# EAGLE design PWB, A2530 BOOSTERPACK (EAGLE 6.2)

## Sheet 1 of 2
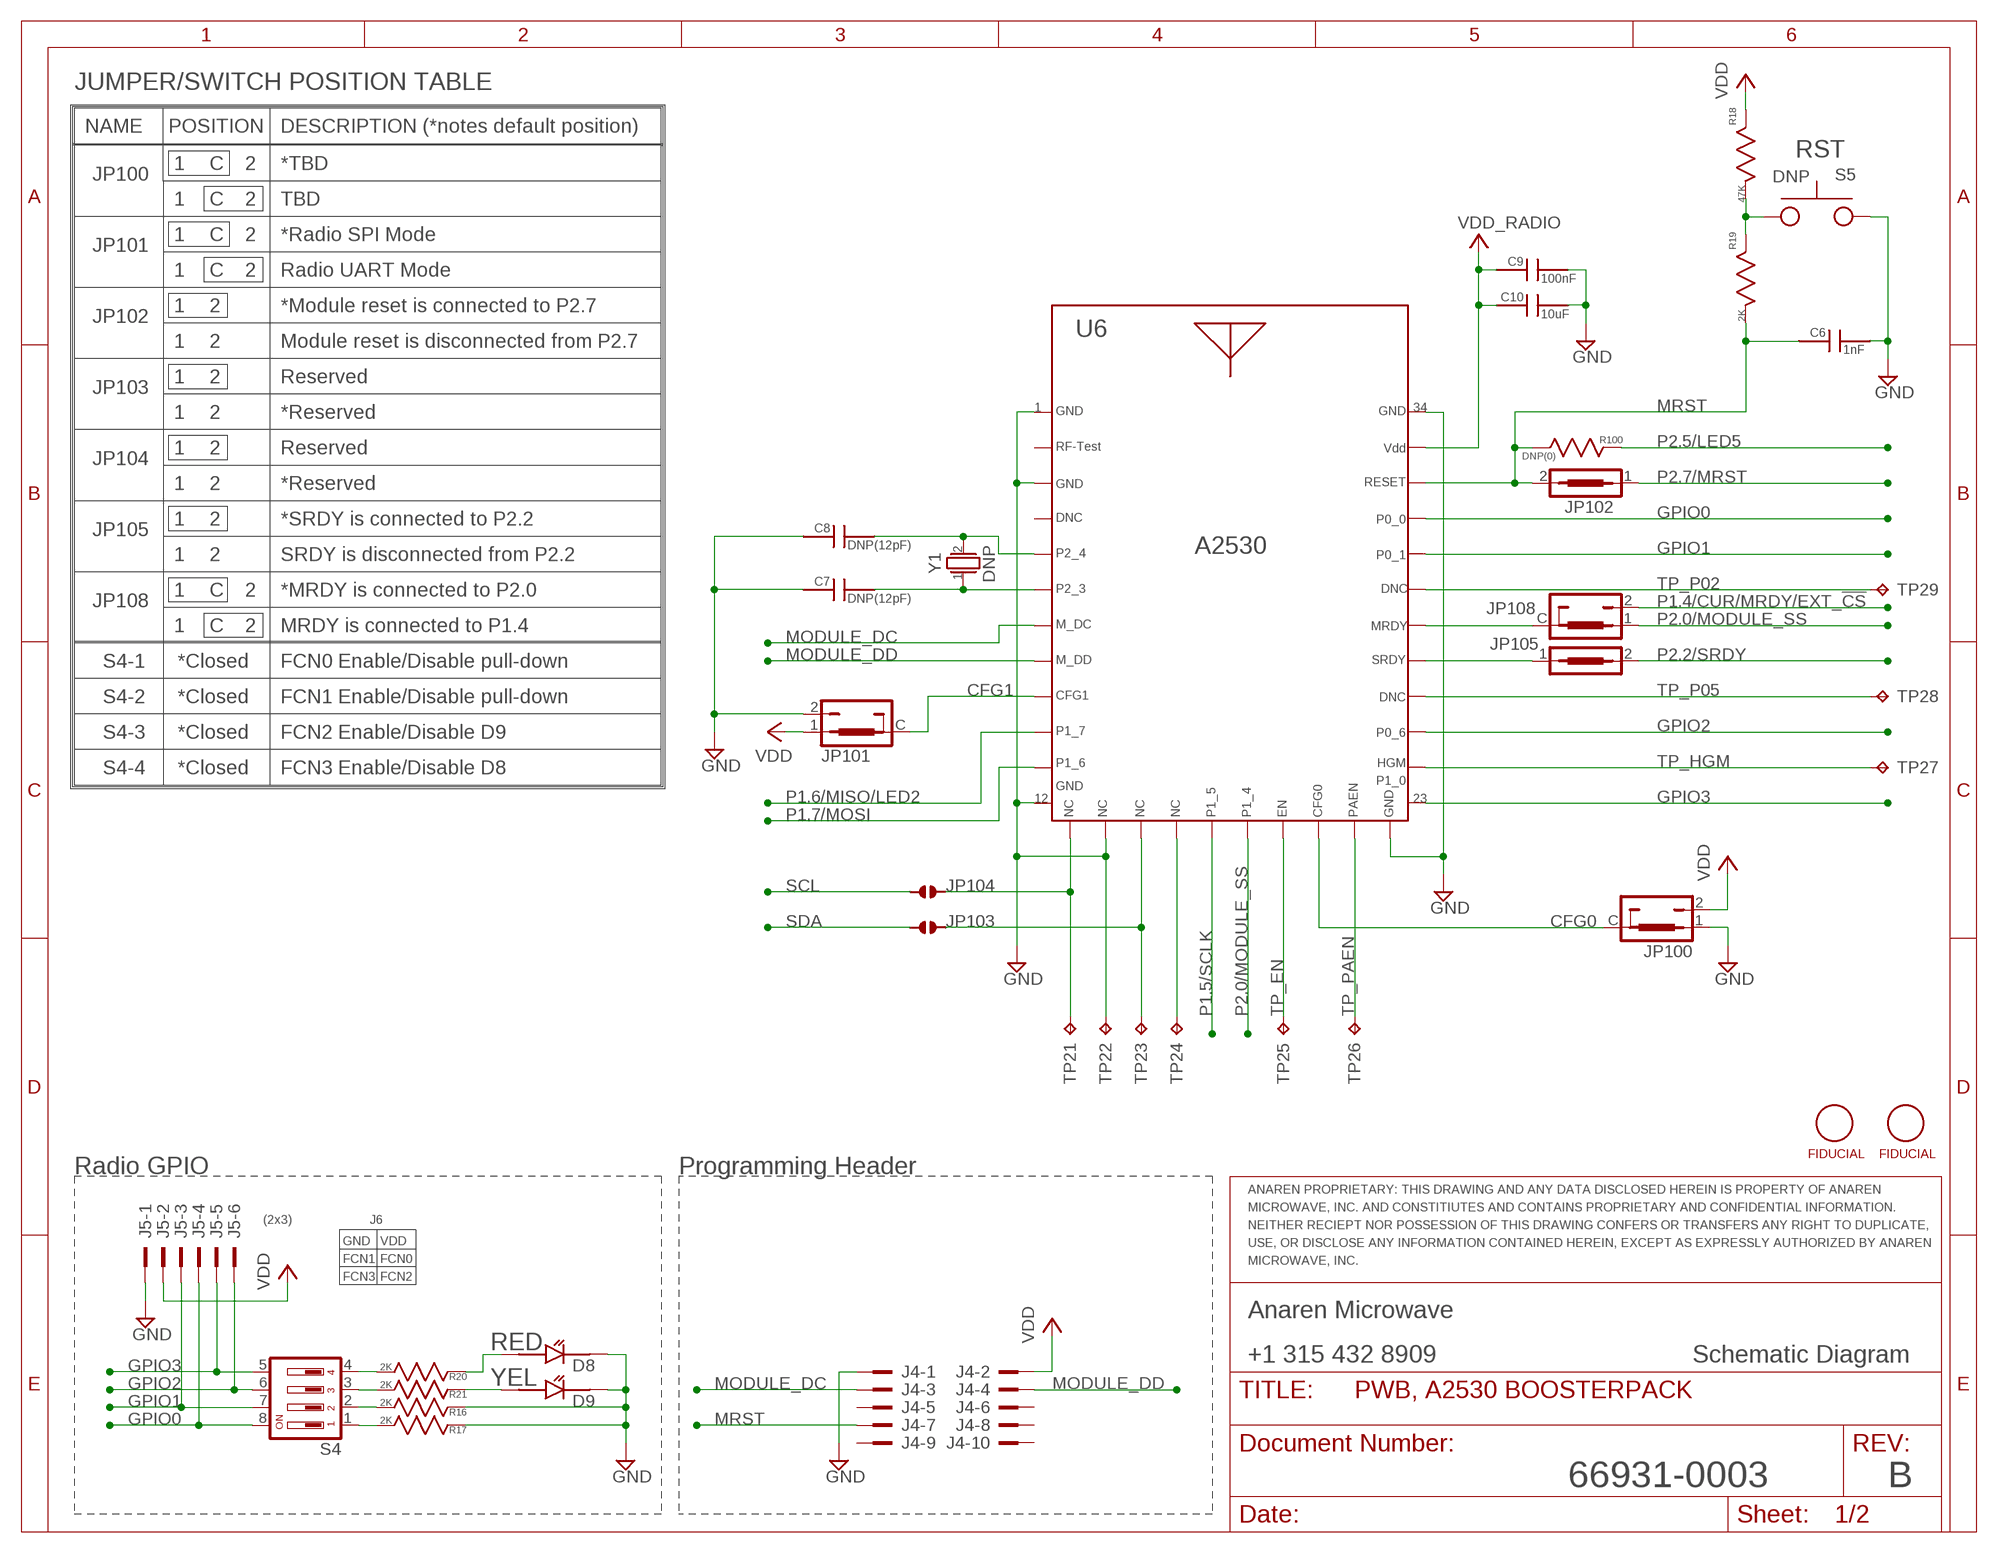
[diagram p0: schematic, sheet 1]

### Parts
C6  1nF  CAP_SMT0402  [0402CAP]
C7  DNP(12pF)  CAP_SMT0402  [0402CAP]
C8  DNP(12pF)  CAP_SMT0402  [0402CAP]
C9  100nF  CAP_SMT0402  [0402CAP]
C10  10uF  CAP_SMT0402  [0402CAP]
D8  LED_SMT_0402  [0402_LED]
D9  LED_SMT_0402  [0402_LED]
J4  SAMTEC_SHF-105-01-L-D-TH_NO_SHROUD  [SAMTEC_SHF-105-01-L-D-TH_NO_SHROUD]
J5  PROTO_100MIL_2X3  [PROTO_100MIL_2X3]
JP100  JP0603_2C_A  [JP0603_2C_A]
JP101  JP0603_2C_A  [JP0603_2C_A]
JP102  JP0603_1P_A  [JP0603_1P_A]
JP103  SOLDER_JUMPER_16MIL  [SOLDER_JUMP_16MIL]
JP104  SOLDER_JUMPER_16MIL  [SOLDER_JUMP_16MIL]
JP105  JP0603_1P_A  [JP0603_1P_A]
JP108  JP0603_2C_A  [JP0603_2C_A]
R16  2K  R0402  [RESC1005X40N]
R17  2K  R0402  [RESC1005X40N]
R18  47K  R0402  [RESC1005X40N]
R19  2K  R0402  [RESC1005X40N]
R20  2K  R0402  [RESC1005X40N]
R21  2K  R0402  [RESC1005X40N]
R100  DNP(0)  0603RES  [0603_COMPONENT]
S4  DIP_SWITCH_218-4LPSTJ  [DIP_SWITCH_218-4LPSTJ]
S5  DNP  SWITCH_B3U-1000P  [SWITCH_B3U-1000P]
TP21  TP_TH_20MIL_R  [TP_TH_20MIL_R]
TP22  TP_TH_20MIL_R  [TP_TH_20MIL_R]
TP23  TP_TH_20MIL_R  [TP_TH_20MIL_R]
TP24  TP_TH_20MIL_R  [TP_TH_20MIL_R]
TP25  TP_TH_20MIL_R  [TP_TH_20MIL_R]
TP26  TP_TH_20MIL_R  [TP_TH_20MIL_R]
TP27  TP_TH_20MIL_R  [TP_TH_20MIL_R]
TP28  TP_TH_20MIL_R  [TP_TH_20MIL_R]
TP29  TP_TH_20MIL_R  [TP_TH_20MIL_R]
U6  CC2530  [CC2530]
U$1  FIDUCIAL0.5MM  [FIDUCIAL_0.5MM]
U$13  FIDUCIAL0.5MM  [FIDUCIAL_0.5MM]
Y1  DNP  ABRACON_ABS06  [ABRACON_ABS06]

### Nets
CFG0: JP100.C U6.20_GIO2
CFG1: JP101.C U6.9_GIO13
GND [GND]: C6.P$2 C7.P$1 C8.P$1 C9.P$2 C10.P$2 D8.2 D9.2 J4.1 J5.1 JP100.1 JP101.2 R16.1 R17.1 S5.2 TP22.P$1(TP) U6.1_GND U6.3_GND U6.12_GND U6.14_USBP U6.22_GND U6.34_GND ; also sheet 2
GPIO0: J5.4 S4.8 U6.31_HGM
GPIO1: J5.3 S4.7 U6.30_GND
GPIO2: J5.6 S4.6 U6.25_BCLK
GPIO3: J5.5 S4.5 U6.23_RSTN
MODULE_DC: J4.3 U6.7_SDA
MODULE_DD: J4.4 U6.8_GIO12
MRDY: JP108.C U6.28_AD1
MRST: C6.P$1 J4.7 JP102.2 R19.2 R100.1 U6.32_IOVDD ; also sheet 2
N$1: R20.2 S4.4
N$2: R21.2 S4.3
N$3: R16.2 S4.2
N$4: R17.2 S4.1
N$5: C7.P$2 U6.6_SCL Y1.1
N$14: D9.1 R21.1
N$15: D8.1 R20.1
N$16: JP104.P2 TP21.P$1(TP) U6.13_USBM
N$17: JP103.P2 TP23.P$1(TP) U6.15_CSN
N$18: R18.2 R19.1 S5.1
N$40: TP24.P$1(TP) U6.16_SCLK
P1.4/CUR/MRDY/EXT_!CS: JP108.2 ; also sheet 2
P1.5/SCLK: U6.17_MOSI ; also sheet 2
P1.6/MISO/LED2: U6.10_PA ; also sheet 2
P1.6/MISO/SCL/LED1: C8.P$2 U6.5_VBAT Y1.2
P1.7/MOSI: U6.11_LNA ; also sheet 2
P2.0/MODULE_SS: JP108.1 U6.18_MISO ; also sheet 2
P2.2/SRDY: JP105.2 ; also sheet 2
P2.5/LED5: R100.2 ; also sheet 2
P2.7/MRST: JP102.1 ; also sheet 2
SCL: JP104.P1 ; also sheet 2
SDA: JP103.P1 ; also sheet 2
SRDY: JP105.1 U6.27_AD0 ; also sheet 2
TP_EN: TP25.P$1(TP) U6.19_GIO1
TP_HGM: TP27.P$1(TP) U6.24_MCLK
TP_P02: TP29.P$1(TP) U6.29_GIO9/AD2
TP_P05: TP28.P$1(TP) U6.26_WCLK
TP_PAEN: TP26.P$1(TP) U6.21_GIO3
VDD [PWR]: J4.2 J5.2 JP100.2 JP101.1 R18.1 ; also sheet 2
VDD_RADIO: C9.P$1 C10.P$1 U6.33_VDD ; also sheet 2
Unconnected: J4.5 J4.6 J4.8 J4.9 J4.10 U6.2_RF_TEST U6.4_DNC

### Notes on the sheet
- JUMPER/SWITCH POSITION TABLE
- NAME | POSITION | DESCRIPTION (*notes default position)
- RST
- 1 | C | 2 | *TBD
- JP100
- 1 | C | 2 | TBD
- 1 | C | 2 | *Radio SPI Mode
- JP101
- 1 | C | 2 | Radio UART Mode
- 1 | 2 | *Module reset is connected to P2.7
- JP102
- 1 | 2 | Module reset is disconnected from P2.7
- 1 | 2 | Reserved
- JP103
- 1 | 34
- 1 | 2 | *Reserved
- 1 | 2 | Reserved
- JP104
- 1 | 2 | *Reserved
- 1 | 2 | *SRDY is connected to P2.2
- JP105
- A2530
- 1 | 2 | SRDY is disconnected from P2.2
- 1 | C | 2 | *MRDY is connected to P2.0
- JP108
- 1 | C | 2 | MRDY is connected to P1.4
- S4-1 | *Closed | FCN0 Enable/Disable pull-down
- S4-2 | *Closed | FCN1 Enable/Disable pull-down
- S4-3 | *Closed | FCN2 Enable/Disable D9
- S4-4 | *Closed | FCN3 Enable/Disable D8
- 12 | 23
- Radio GPIO | Programming Header
- ANAREN PROPRIETARY: THIS DRAWING AND ANY DATA DISCLOSED HEREIN IS PROPERTY OF ANAREN
- MICROWAVE, INC. AND CONSTITIUTES AND CONTAINS PROPRIETARY AND CONFIDENTIAL INFORMATION.
- (2x3) | J6
- NEITHER RECIEPT NOR POSSESSION OF THIS DRAWING CONFERS OR TRANSFERS ANY RIGHT TO DUPLICATE,
- GND | VDD | USE, OR DISCLOSE ANY INFORMATION CONTAINED HEREIN, EXCEPT AS EXPRESSLY AUTHORIZED BY ANAREN
- FCN1 | FCN0 | MICROWAVE, INC.
- FCN3 | FCN2
- Anaren Microwave
- RED
- +1 315 432 8909 | Schematic Diagram
- YEL
- 66931-0003 | B

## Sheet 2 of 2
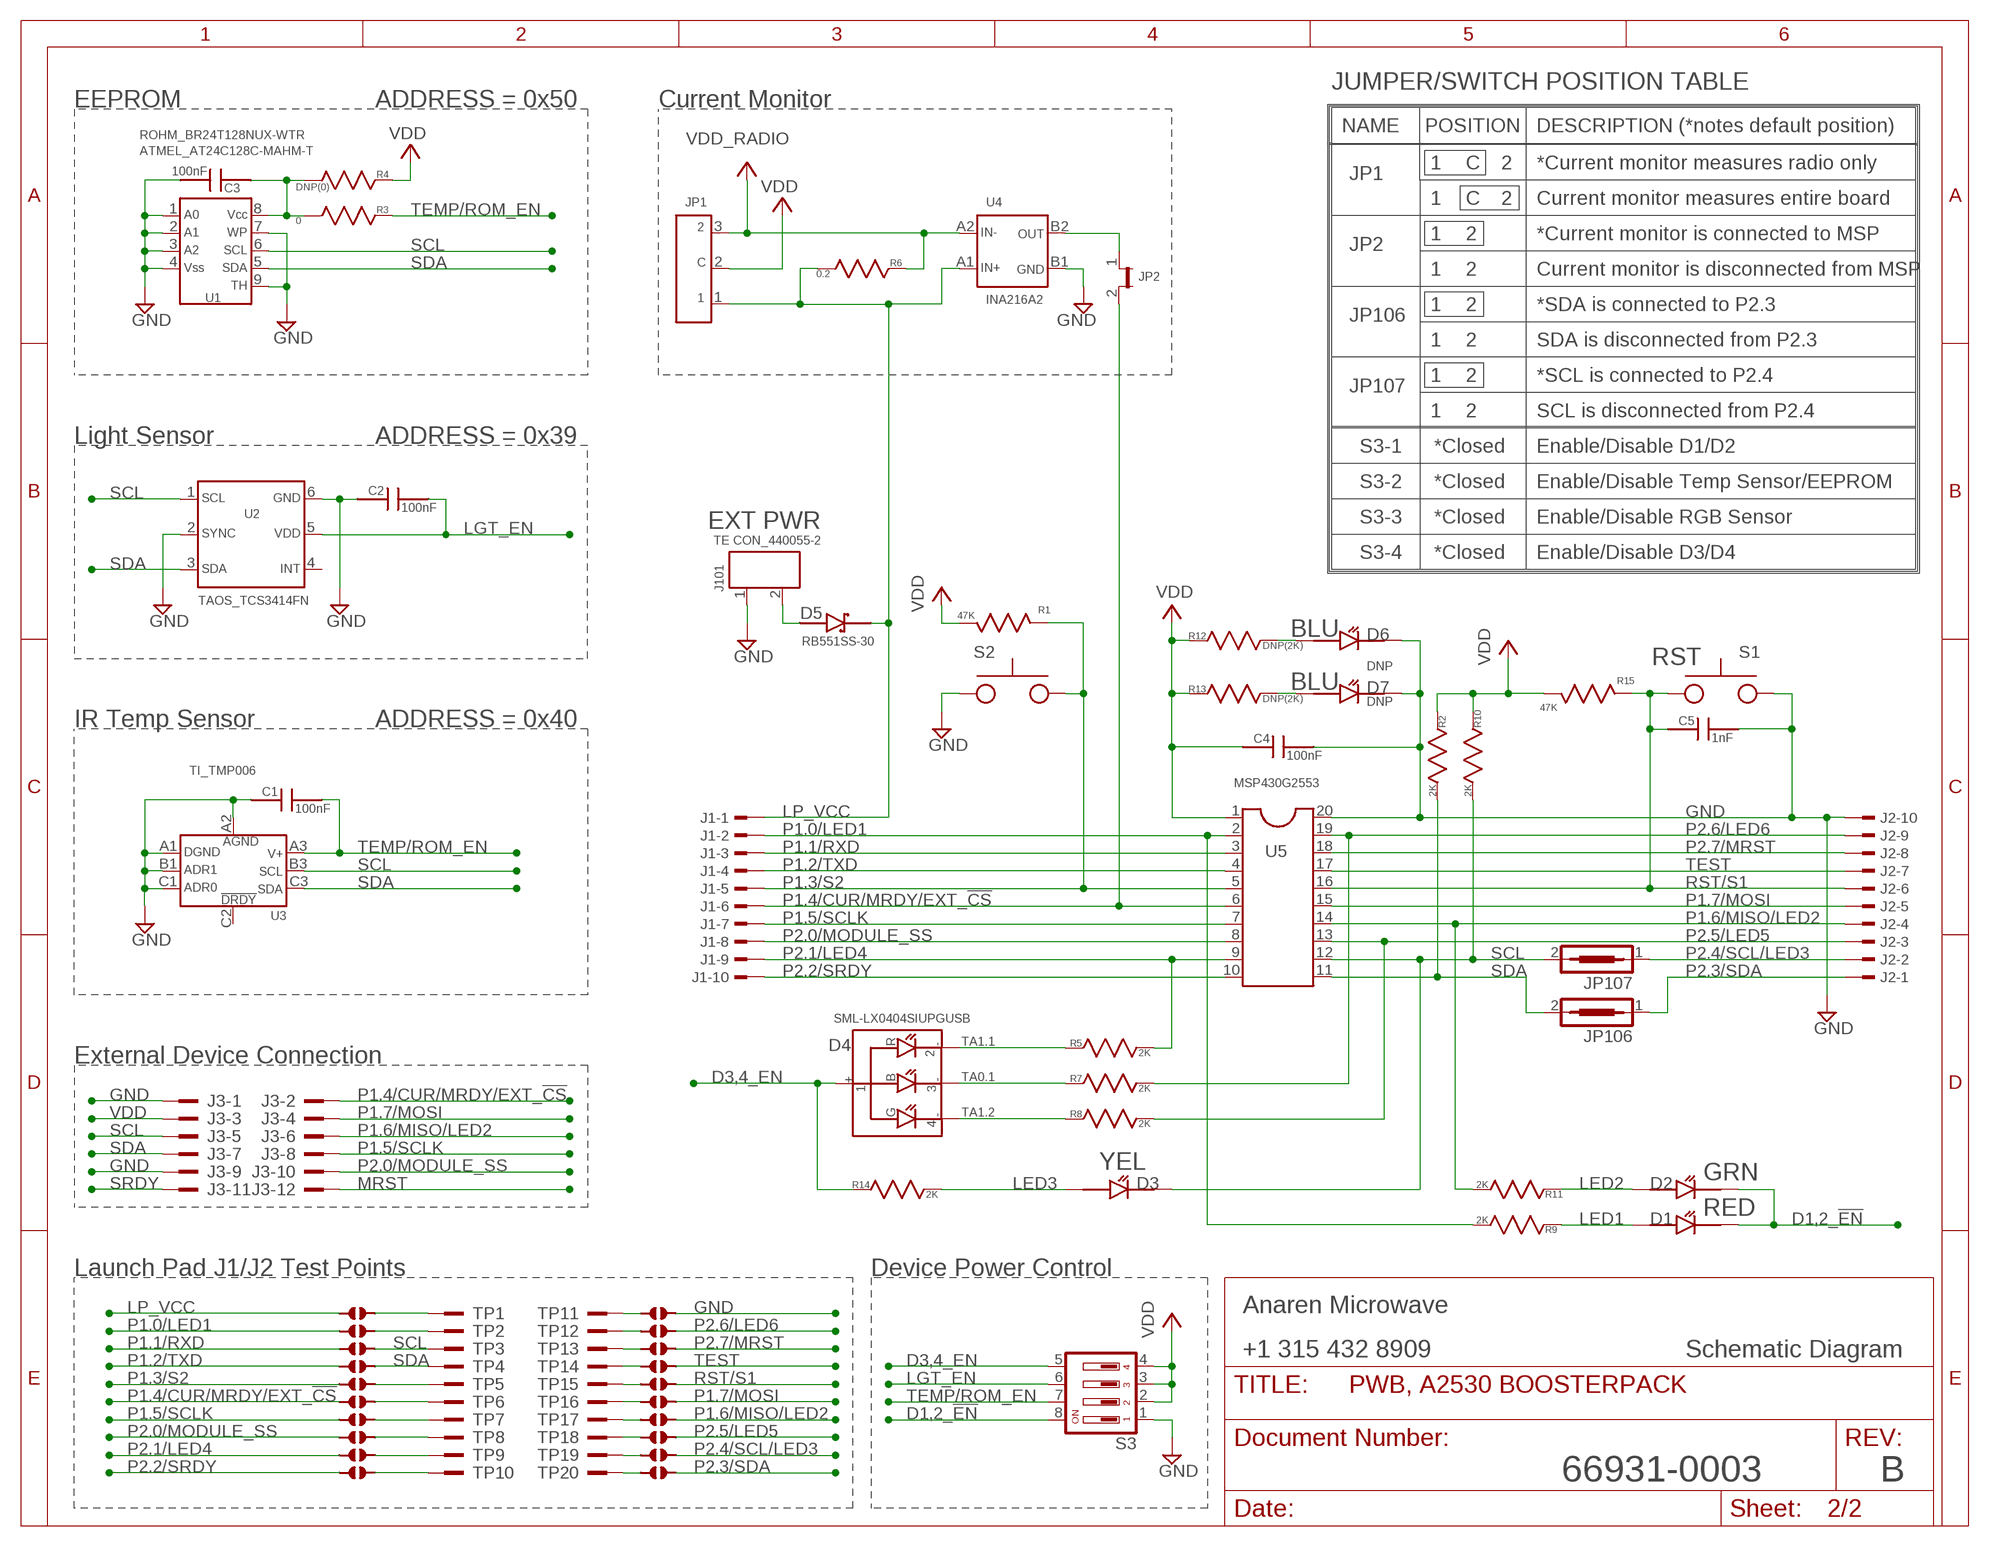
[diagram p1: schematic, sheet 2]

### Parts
C1  100nF  CAP_SMT0402  [0402CAP]
C2  100nF  CAP_SMT0402  [0402CAP]
C3  100nF  CAP_SMT0402  [0402CAP]
C4  100nF  CAP_SMT0402  [0402CAP]
C5  1nF  CAP_SMT0402  [0402CAP]
D1  LED_SMT_0402  [0402_LED]
D2  LED_SMT_0402  [0402_LED]
D3  LED_SMT_0402  [0402_LED]
D4  SML-LX0404SIUPGUSB  [SML-LXO404SIUPGUSB]
D5  RB551SS-30  [1608_DIODE]
D6  LED_SMT_0402  [0402_LED]
D7  LED_SMT_0402  [0402_LED]
J1  TSW-110-02-S-S  [TSW-110-02-S-S]
J2  TSW-110-02-S-S  [TSW-110-02-S-S]
J3  PROTO_100MIL_2X6  [PROTO_100MIL_2X6]
J101  TE_CONNECTIVITY_HEADER_2POS_2MM_RIGHT_ANGLE_T/H  [TE_CONNECTIVITY_HEADER_2POS_2MM_RIGHT_ANGLE_TH]
JP1  SAMTEC_TMM-103-XX-X-S  [SAMTEC_TMM-103-XX-X-S]
JP2  2MM_SHUNT_JUMPER  [SAMTEC_TMM-102-XX-X-S]
JP106  JP0603_1P_A  [JP0603_1P_A]
JP107  JP0603_1P_A  [JP0603_1P_A]
R1  47K  R0402  [RESC1005X40N]
R2  2K  R0402  [RESC1005X40N]
R3  0  R0402  [RESC1005X40N]
R4  DNP(0)  R0402  [RESC1005X40N]
R5  2K  R0402  [RESC1005X40N]
R6  0.2  R0402  [RESC1005X40N]
R7  2K  R0402  [RESC1005X40N]
R8  2K  R0402  [RESC1005X40N]
R9  2K  R0402  [RESC1005X40N]
R10  2K  R0402  [RESC1005X40N]
R11  2K  R0402  [RESC1005X40N]
R12  DNP(2K)  R0402  [RESC1005X40N]
R13  DNP(2K)  R0402  [RESC1005X40N]
R14  2K  R0402  [RESC1005X40N]
R15  47K  R0402  [RESC1005X40N]
S1  SWITCH_B3U-1000P  [SWITCH_B3U-1000P]
S2  SWITCH_B3U-1000P  [SWITCH_B3U-1000P]
S3  DIP_SWITCH_218-4LPSTJ  [DIP_SWITCH_218-4LPSTJ]
TP1  PROTO  [PROTO]
TP2  PROTO  [PROTO]
TP3  PROTO  [PROTO]
TP4  PROTO  [PROTO]
TP5  PROTO  [PROTO]
TP6  PROTO  [PROTO]
TP7  PROTO  [PROTO]
TP8  PROTO  [PROTO]
TP9  PROTO  [PROTO]
TP10  PROTO  [PROTO]
TP11  PROTO  [PROTO]
TP12  PROTO  [PROTO]
TP13  PROTO  [PROTO]
TP14  PROTO  [PROTO]
TP15  PROTO  [PROTO]
TP16  PROTO  [PROTO]
TP17  PROTO  [PROTO]
TP18  PROTO  [PROTO]
TP19  PROTO  [PROTO]
TP20  PROTO  [PROTO]
U1  ROHM_BR24T128NUX-WTR  [UFDFN8_2.0X3.0]
U2  TAOS_TCS3414FN  [TAOS_DFP_3.5X2.3]
U3  TI_TMP006  [BGA-N8]
U4  INA216A2  [WCSP-4]
U5  DIL20  [DIL20]
U$2  SOLDER_JUMPER_16MIL  [SOLDER_JUMP_16MIL]
U$3  SOLDER_JUMPER_16MIL  [SOLDER_JUMP_16MIL]
U$4  SOLDER_JUMPER_16MIL  [SOLDER_JUMP_16MIL]
U$5  SOLDER_JUMPER_16MIL  [SOLDER_JUMP_16MIL]
U$6  SOLDER_JUMPER_16MIL  [SOLDER_JUMP_16MIL]
U$7  SOLDER_JUMPER_16MIL  [SOLDER_JUMP_16MIL]
U$8  SOLDER_JUMPER_16MIL  [SOLDER_JUMP_16MIL]
U$9  SOLDER_JUMPER_16MIL  [SOLDER_JUMP_16MIL]
U$10  SOLDER_JUMPER_16MIL  [SOLDER_JUMP_16MIL]
U$11  SOLDER_JUMPER_16MIL  [SOLDER_JUMP_16MIL]
U$14  SOLDER_JUMPER_16MIL  [SOLDER_JUMP_16MIL]
U$15  SOLDER_JUMPER_16MIL  [SOLDER_JUMP_16MIL]
U$16  SOLDER_JUMPER_16MIL  [SOLDER_JUMP_16MIL]
U$17  SOLDER_JUMPER_16MIL  [SOLDER_JUMP_16MIL]
U$18  SOLDER_JUMPER_16MIL  [SOLDER_JUMP_16MIL]
U$19  SOLDER_JUMPER_16MIL  [SOLDER_JUMP_16MIL]
U$20  SOLDER_JUMPER_16MIL  [SOLDER_JUMP_16MIL]
U$21  SOLDER_JUMPER_16MIL  [SOLDER_JUMP_16MIL]
U$22  SOLDER_JUMPER_16MIL  [SOLDER_JUMP_16MIL]
U$23  SOLDER_JUMPER_16MIL  [SOLDER_JUMP_16MIL]

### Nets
CURRENT: JP2.1 U4.B2
D1,2_!EN [GND]: D1.2 D2.2 S3.8
D3,4_EN: D4.1(+) R14.1 S3.5
GND [GND]: C1.P$1 C2.P$1 C3.P$2 C4.P$2 C5.P$2 D6.2 D7.2 J2.10 J3.1 J3.9 J101.1 S1.2 S2.2 S3.1 U1.1 U1.2 U1.3 U1.4 U1.7 U1.9 U2.2 U2.6 U3.A1 U3.A2 U3.B1 U3.C1 U4.B1 U5.20 U$14.P2 ; also sheet 1
LED1: D1.1 R9.1
LED2: D2.1 R11.1
LED3: D3.1 R14.2
LED4: D4.2(-R) R5.1
LED5: D4.4(-G) R8.1
LED6: D4.3(-B) R7.1
LGT_EN [PWR]: C2.P$2 S3.6 U2.5
LP_VCC [PWR]: D5.P$2 J1.1 JP1.1 R6.2 U4.A1 U$2.P1
MRST: J3.12 ; also sheet 1
N$6: D6.1 R12.2
N$7: D7.1 R13.2
N$11: C3.P$1 R3.2 R4.2 U1.8
N$19 [PWR]: TP1.1(KL) U$2.P2
N$24: TP5.1(KL) U$6.P2
N$25: TP6.1(KL) U$7.P2
N$26: TP7.1(KL) U$8.P2
N$27: TP8.1(KL) U$9.P2
N$28: TP9.1(KL) U$10.P2
N$29: TP10.1(KL) U$11.P2
N$30 [GND]: TP11.1(KL) U$14.P1
N$31: TP12.1(KL) U$15.P1
N$32: TP13.1(KL) U$16.P1
N$33: TP14.1(KL) U$17.P1
N$34: TP15.1(KL) U$18.P1
N$35: TP16.1(KL) U$19.P1
N$36: TP17.1(KL) U$20.P1
N$37: TP18.1(KL) U$21.P1
N$38: TP19.1(KL) U$22.P1
N$39: TP20.1(KL) U$23.P1
N$42 [PWR]: D5.P$1 J101.2
P1.0/LED1: J1.2 R9.2 U5.2 U$3.P1
P1.1/RXD: J1.3 U5.3 U$4.P1
P1.2/TXD: J1.4 U5.4 U$5.P1
P1.3/S2: J1.5 R1.1 S2.1 U5.5 U$6.P1
P1.4/CUR/MRDY/EXT_!CS: J1.6 J3.2 JP2.2 U5.6 U$7.P1 ; also sheet 1
P1.5/SCLK: J1.7 J3.8 U5.7 U$8.P1 ; also sheet 1
P1.6/MISO/LED2: J2.4 J3.6 R11.2 U5.14 U$20.P2 ; also sheet 1
P1.7/MOSI: J2.5 J3.4 U5.15 U$19.P2 ; also sheet 1
P2.0/MODULE_SS: J1.8 J3.10 U5.8 U$9.P1 ; also sheet 1
P2.1/LED4: J1.9 R5.2 U5.9 U$10.P1
P2.2/SRDY: J1.10 U5.10 U$11.P1 ; also sheet 1
P2.3/SDA: J2.1 JP106.1 U$23.P2
P2.4/SCL/LED3: J2.2 JP107.1 U$22.P2
P2.5/LED5: J2.3 R8.2 U5.13 U$21.P2 ; also sheet 1
P2.6/LED6: J2.9 R7.2 U5.19 U$15.P2
P2.7/MRST: J2.8 U5.18 U$16.P2 ; also sheet 1
RST/S1: C5.P$1 J2.6 R15.1 S1.1 U5.16 U$18.P2
SCL: D3.2 J3.5 JP107.2 R10.2 TP3.1(KL) U1.6 U2.1 U3.B3 U5.12 U$4.P2 ; also sheet 1
SDA: J3.7 JP106.2 R2.2 TP4.1(KL) U1.5 U2.3 U3.C3 U5.11 U$5.P2 ; also sheet 1
SRDY: J3.11 ; also sheet 1
STLRS_GND [PWR]: TP2.1(KL) U$3.P2
TEMP/ROM_EN [PWR]: C1.P$2 R3.1 S3.7 U3.A3
TEST: J2.7 U5.17 U$17.P2
VDD [PWR]: C4.P$1 J3.3 JP1.2 R1.2 R2.1 R4.1 R10.1 R12.1 R13.1 R15.2 S3.2 S3.3 S3.4 U5.1 ; also sheet 1
VDD_RADIO: JP1.3 R6.1 U4.A2 ; also sheet 1
Unconnected: U2.4 U3.C2

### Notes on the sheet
- JUMPER/SWITCH POSITION TABLE
- EEPROM | ADDRESS = 0x50 | Current Monitor
- NAME | POSITION | DESCRIPTION (*notes default position)
- ATMEL_AT24C128C-MAHM-T
- 1 | C | 2 | *Current monitor measures radio only
- JP1
- 1 | C | 2 | Current monitor measures entire board
- 2
- 1 | 2 | *Current monitor is connected to MSP
- JP2
- C
- 1 | 2 | Current monitor is disconnected from MSP
- 1
- 1 | 2 | *SDA is connected to P2.3
- JP106
- 1 | 2 | SDA is disconnected from P2.3
- 1 | 2 | *SCL is connected to P2.4
- JP107
- 1 | 2 | SCL is disconnected from P2.4
- Light Sensor | ADDRESS = 0x39
- S3-1 | *Closed | Enable/Disable D1/D2
- S3-2 | *Closed | Enable/Disable Temp Sensor/EEPROM
- EXT PWR | S3-3 | *Closed | Enable/Disable RGB Sensor
- TE CON_440055-2
- S3-4 | *Closed | Enable/Disable D3/D4
- BLU
- RST
- DNP
- BLU
- DNP
- IR Temp Sensor | ADDRESS = 0x40
- MSP430G2553
- TA1.1
- External Device Connection
- TA0.1
- TA1.2
- YEL
- GRN
- RED
- Launch Pad J1/J2 Test Points | Device Power Control
- Anaren Microwave
- +1 315 432 8909 | Schematic Diagram
- 66931-0003 | B

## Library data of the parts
C1-C10 = Anaren_2:CAP_SMT
D1-D3 D6-D9 = Anaren_2:LED_SMT_0402
D4 = Anaren_2:SML-LX0404SIUPGUSB
D5 = Anaren_2:RB551SS-30
J1 J2 = con-samtec:TSW-110-02-S-S: THROUGH-HOLE .025" SQ POST HEADER Source: Samtec TSW.pdf; OC_FARNELL: unknown; OC_NEWARK: unknown
J3 = Anaren_2:PROTO_100MIL_2X6
J4 = Anaren_2:SAMTEC_SHF-105-01-L-D-TH_NO_SHROUD
J5 = Anaren_2:PROTO_100MIL_2X3
J101 = Anaren_2:TE_CONNECTIVITY_HEADER_2POS_2MM_RIGHT_ANGLE_T/H
JP1 = Anaren_2:SAMTEC_TMM-103-XX-X-S
JP2 = Anaren_2:2MM_SHUNT_JUMPER
JP100 JP101 JP108 = Anaren_MGS:JP0603_2C_A
JP102 JP105-JP107 = Anaren_MGS:JP0603_1P_A
JP103 JP104 U$2-U$11 U$14-U$23 = Anaren_2:SOLDER_JUMPER_16MIL
R1-R21 = Anaren_MGS:R0402
R100 = Anaren_2:0603RES
S1 S2 S5 = Anaren_MGS:SWITCH_B3U-1000P: 1.2 X 3.0mm TACT Switch (SMD)
S3 S4 = Anaren_2:DIP_SWITCH_218-4LPSTJ
TP1-TP20 = Anaren_2:PROTO
TP21-TP29 = Anaren_2:TP_TH_20MIL_R
U1 = Anaren_2:ROHM_BR24T128NUX-WTR
U2 = Anaren_2:TAOS_TCS3414FN
U3 = Anaren_2:TI_TMP006
U4 = Anaren_2:INA216A2
U5 = ic-package:DIL20: Dual In Line / Socket
U6 = Anaren_2:CC2530
U$1 U$13 = Anaren_MGS:FIDUCIAL
Y1 = Anaren_2:ABRACON_ABS06

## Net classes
0 default: clearance 0.127 mm
1 GND: clearance 0.203 mm
2 RF: width 0.516 mm, clearance 0.635 mm
3 PWR: clearance 0.203 mm

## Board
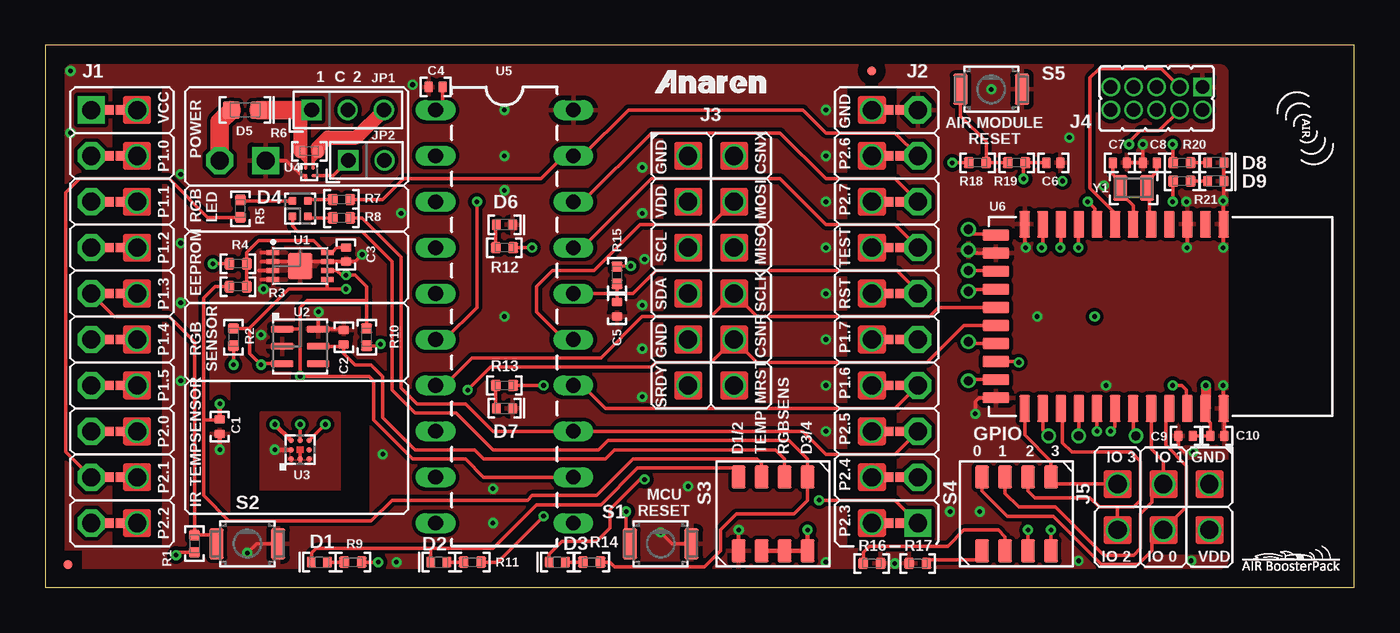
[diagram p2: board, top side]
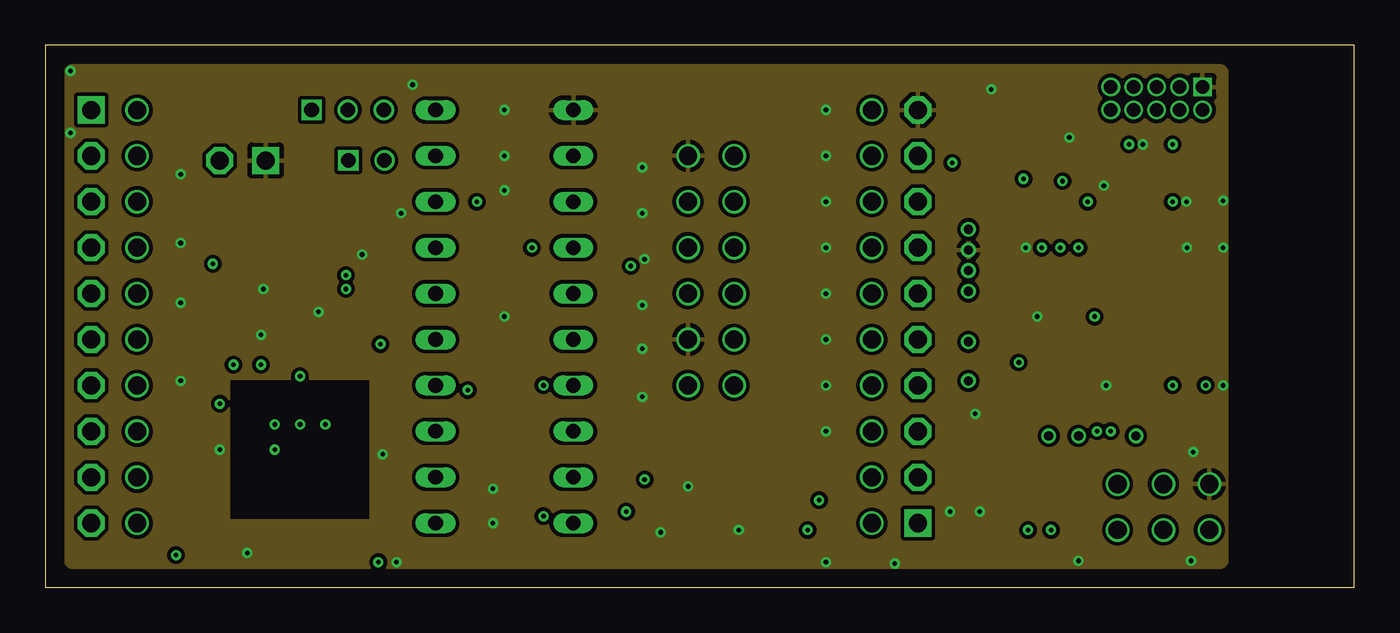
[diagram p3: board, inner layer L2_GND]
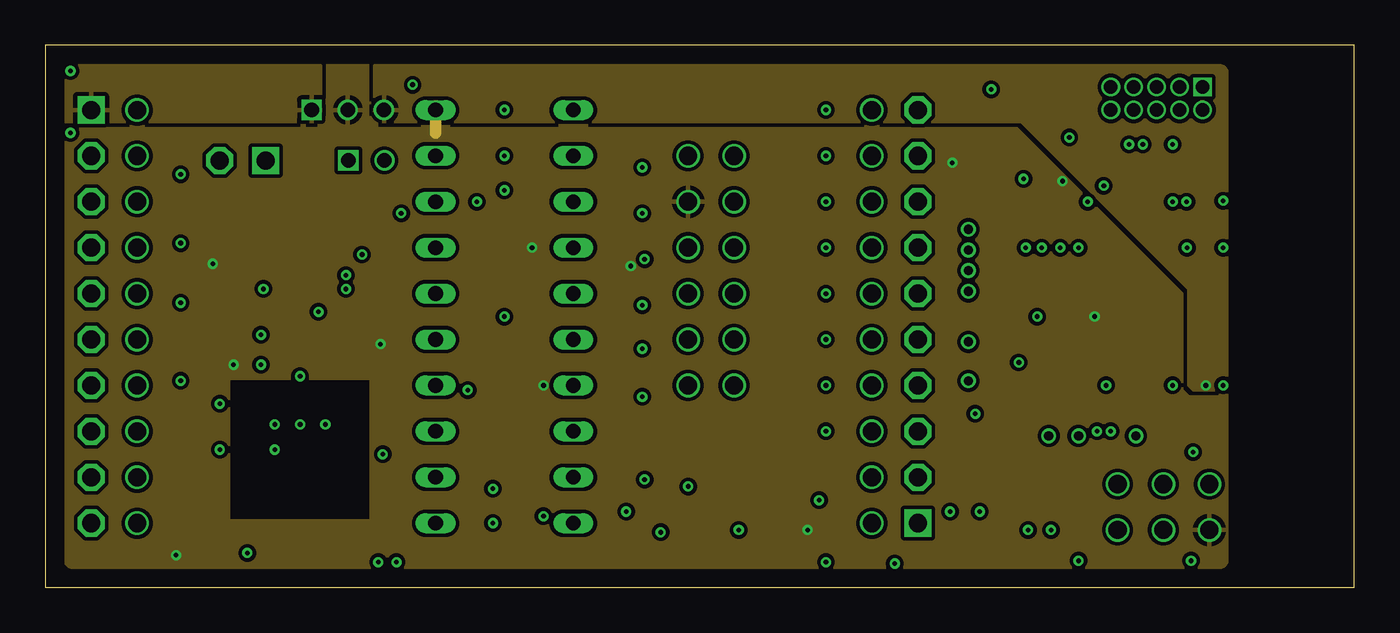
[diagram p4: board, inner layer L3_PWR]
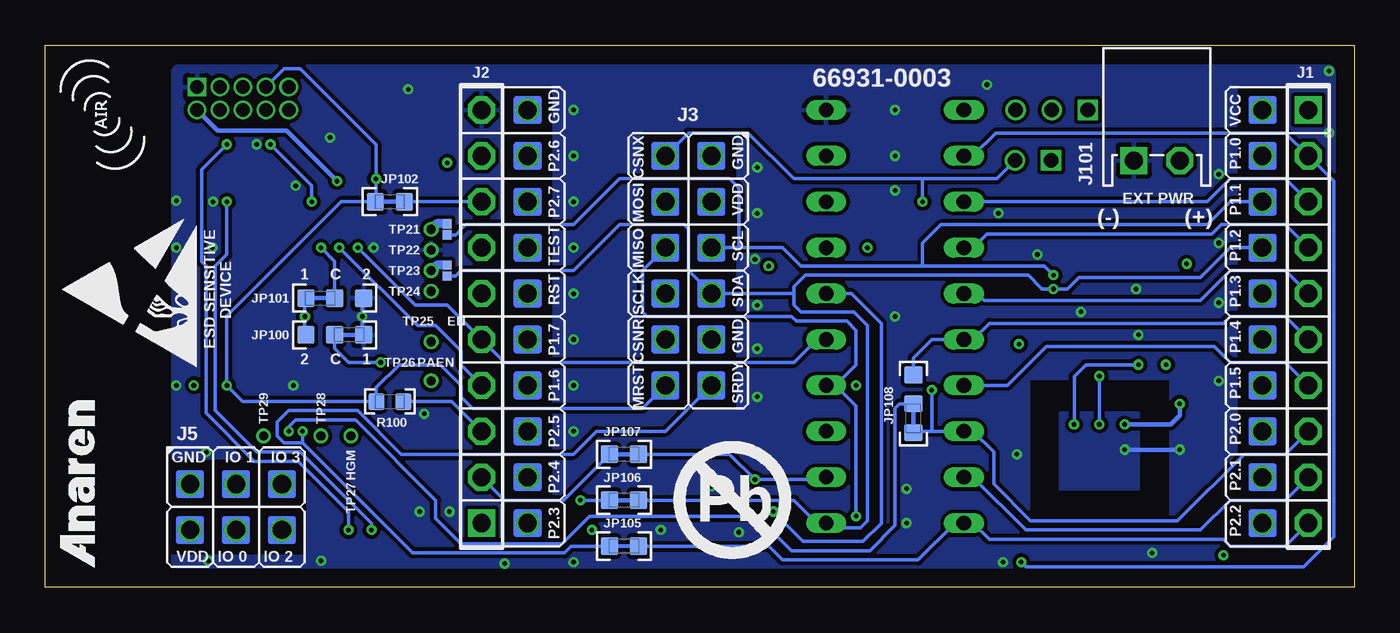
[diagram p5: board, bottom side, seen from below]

Size 72.4 x 30 mm. Coordinates in mm from the lower left corner, seen from the top.
Outline: 0,0 72.4,0 72.4,30 0,30 0,0
Copper layers ((1*2)+(15*16)): Top 0.0175mm / dielectric 5mil / L2_GND 0.0175mm / dielectric 50mil / L3_PWR 0.0175mm / dielectric 5mil / Bottom 0.0175mm
Design rules: minimum track width 5mil, minimum drill 10mil, track to track 8mil, track to pad 8mil, pad to pad 8mil, via to via 8mil, smd to smd 0.1mm, copper to edge 40mil, drill to drill 8mil, minimum pad ring 6mil, minimum via ring 6mil, stop-mask expansion 4mil, vias tented up to drill 10mil, thermal gap 10mil
tRestrict: area 0.5,0.5 to 2,2; area 13.6,7.1 to 14.6,8.1; area 65.5,0.5 to 71.9,29.5
bRestrict: area 65.5,0.5 to 71.9,29.5

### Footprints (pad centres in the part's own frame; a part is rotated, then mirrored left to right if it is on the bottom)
0402CAP = smd 0.483 x 0.61: P$1 -0.394,0; P$2 0.394,0
0402_LED = smd 0.5 x 0.6: 1 -0.45,0; 2 0.45,0
SML-LXO404SIUPGUSB = smd 0.45 x 0.45: 1(+) 0.425,0.425; 2(-R) 0.425,-0.425; 3(-B) -0.425,-0.425; 4(-G) -0.425,0.425
1608_DIODE = smd 0.9 x 0.95: P$1 -0.75,0; P$2 0.75,0
TSW-110-02-S-S = drill 1 pad 1.5 square: 1 11.43,0 | drill 1 pad 1.5 octagon: 2 8.89,0; 3 6.35,0; 4 3.81,0; 5 1.27,0; 6 -1.27,0; 7 -3.81,0; 8 -6.35,0; 9 -8.89,0; 10 -11.43,0
PROTO_100MIL_2X6 = drill 1: 1 0,0; 2 2.54,0; 3 0,-2.54; 4 2.54,-2.54; 5 0,-5.08; 6 2.54,-5.08; 7 0,-7.62; 8 2.54,-7.62; 9 0,-10.16; 10 2.54,-10.16; 11 0,-12.7; 12 2.54,-12.7
SAMTEC_SHF-105-01-L-D-TH_NO_SHROUD = drill 0.737 pad 1.041 square: 1 -2.54,-0.635 | drill 0.737 pad 1.041: 2 -2.54,0.635; 3 -1.27,-0.635; 4 -1.27,0.635; 5 0,-0.635; 6 0,0.635; 8 1.27,0.635; 9 2.54,-0.635; 10 2.54,0.635 | drill 0.737 pad 0.991: 7 1.27,-0.635
PROTO_100MIL_2X3 = drill 1: 1 0,0; 2 2.54,0; 3 0,-2.54; 4 2.54,-2.54; 5 0,-5.08; 6 2.54,-5.08
TE_CONNECTIVITY_HEADER_2POS_2MM_RIGHT_ANGLE_TH = drill 1 pad 1.5 square: 1 -1.27,0 | drill 1 pad 1.5 octagon: 2 1.27,0
SAMTEC_TMM-103-XX-X-S = drill 0.813 square: 1 0,0 | drill 0.813: 2 2,0; 3 4,0
SAMTEC_TMM-102-XX-X-S = drill 0.813 square: 1 0,0 | drill 0.813: 2 2,0
JP0603_2C_A = smd 0.95 x 1: 1 -1.6,0; 2 1.6,0; C 0,0
JP0603_1P_A = smd 0.95 x 1: 1 -0.8,0; 2 0.8,0
SOLDER_JUMP_16MIL = smd 0.508 x 0.508: P1 -0.305,0; P2 0.305,0
RESC1005X40N = smd 0.57 x 0.62: 1 -0.48,0; 2 0.48,0
0603_COMPONENT = smd 0.9 x 0.95: 1 -0.75,0; 2 0.75,0
SWITCH_B3U-1000P = smd 0.8 x 1.7: 1 -1.7,0; 2 1.7,0
DIP_SWITCH_218-4LPSTJ = smd 1.27 x 0.762: 1 -2.045,1.905; 2 -2.045,0.635; 3 -2.045,-0.635; 4 -2.045,-1.905; 5 2.045,-1.905; 6 2.045,-0.635; 7 2.045,0.635; 8 2.045,1.905
PROTO = drill 1: 1 0,0
TP_TH_20MIL_R = drill 0.508: P$1 0,0
UFDFN8_2.0X3.0 = smd 0.3 x 0.75: 1 -0.75,-1.5; 2 -0.25,-1.5; 3 0.25,-1.5; 4 0.75,-1.5; 5 0.75,1.5; 6 0.25,1.5; 7 -0.25,1.5; 8 -0.75,1.5 | smd 1.46 x 1.36: 9 0,0
TAOS_DFP_3.5X2.3 = smd 1.25 x 0.4: 1 -1,0.95; 2 -1,0; 3 -1,-0.95; 4 1,-0.95; 5 1,0; 6 1,0.95
BGA-N8 = smd 0.3 x 0.3: A1 -0.5,0.5; A2 0,0.5; A3 0.5,0.5; B1 -0.5,0; B3 0.5,0; C1 -0.5,-0.5; C2 0,-0.5; C3 0.5,-0.5
WCSP-4 = smd 0.2 x 0.2: A1 -0.2,-0.2; A2 -0.2,0.2; B1 0.2,-0.2; B2 0.2,0.2
DIL20 = drill 0.813 long: 1 -11.43,-3.81; 2 -8.89,-3.81; 3 -6.35,-3.81; 4 -3.81,-3.81; 5 -1.27,-3.81; 6 1.27,-3.81; 7 3.81,-3.81; 8 6.35,-3.81; 9 8.89,-3.81; 10 11.43,-3.81; 11 11.43,3.81; 12 8.89,3.81; 13 6.35,3.81; 14 3.81,3.81; 15 1.27,3.81; 16 -1.27,3.81; 17 -3.81,3.81; 18 -6.35,3.81; 19 -8.89,3.81; 20 -11.43,3.81
CC2530 = smd 1.499 x 0.61: 1_GND -0.596,12.591; 2_RF_TEST -0.596,11.591; 3_GND -0.596,10.591; 4_DNC -0.596,9.591; 5_VBAT -0.596,8.591; 6_SCL -0.596,7.591; 7_SDA -0.596,6.591; 8_GIO12 -0.596,5.591; 9_GIO13 -0.596,4.591; 10_PA -0.596,3.591; 11_LNA -0.596,2.591; 12_GND -0.596,1.591; 23_RSTN 9.596,1.591; 24_MCLK 9.596,2.591; 25_BCLK 9.596,3.591; 26_WCLK 9.596,4.591; 27_AD0 9.596,5.591; 28_AD1 9.596,6.591; 29_GIO9/AD2 9.596,7.591; 30_GND 9.596,8.591; 31_HGM 9.596,9.591; 32_IOVDD 9.596,10.591; 33_VDD 9.596,11.591; 34_GND 9.596,12.591 | smd 0.61 x 1.499: 13_USBM 0,0; 14_USBP 1,0; 15_CSN 2,0; 16_SCLK 3,0; 17_MOSI 4,0; 18_MISO 5,0; 19_GIO1 6,0; 20_GIO2 7,0; 21_GIO3 8,0; 22_GND 9,0
FIDUCIAL_0.5MM = smd 0.5 x 0.5: P$1 0,0
ABRACON_ABS06 = smd 0.762 x 1.397: 1 -0.737,0; 2 0.737,0

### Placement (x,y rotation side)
C1  9.65,8.89 90 top
C2  16.51,13.84 270 top
C3  16.64,18.41 270 top
C4  21.59,27.69 180 top
C5  31.62,15.39 270 top
C6  55.75,23.5 0 top
C7  59.44,23.5 180 top
C8  61.09,23.5 0 top
C9  63.07,8.38 180 top
C10  64.82,8.38 0 top
D1  15.16,1.4 180 top
D2  21.77,1.4 180 top
D3  28.32,1.4 180 top
D4  14.1,20.95 180 top
D5  11.05,26.42 0 top
D6  25.4,20.07 0 top
D7  25.4,9.91 0 top
D8  64.74,23.5 0 top
D9  64.74,22.48 0 top
DRILEGEND  [DRILEGEND]  not placed on the board
J1  2.54,14.99 90 bottom
J2  48.26,14.99 270 bottom
J3  35.56,23.88 0 top
J4  61.47,27.05 180 top
J5  64.39,5.71 270 top
J101  10.92,23.62 0 bottom
JP1  14.73,26.42 0 top
JP2  16.76,23.62 0 top
JP100  56.39,13.97 180 bottom
JP101  56.39,16 0 bottom
JP102  53.34,21.34 180 bottom
JP103  50.16,17.53 90 bottom
JP104  50.16,19.81 90 bottom
JP105  40.39,2.29 0 bottom
JP106  40.39,4.83 0 bottom
JP107  40.39,7.37 0 bottom
JP108  24.38,10.16 90 bottom
R1  8.26,2.42 270 top
R2  10.41,13.84 90 top
R3  10.67,16.64 0 top
R4  10.67,17.91 0 top
R5  10.79,20.95 270 top
R6  14.61,24.13 180 top
R7  16.38,21.46 0 top
R8  16.38,20.45 0 top
R9  17.02,1.4 0 top
R10  17.78,13.84 90 top
R11  23.62,1.4 0 top
R12  25.4,18.8 180 top
R13  25.4,11.18 180 top
R14  30.23,1.4 180 top
R15  31.62,17.27 90 top
R16  45.72,1.33 180 top
R17  48.26,1.33 0 top
R18  51.56,23.5 0 top
R19  53.72,23.5 0 top
R20  62.87,23.5 180 top
R21  62.87,22.48 180 top
R100  53.34,10.29 0 bottom
S1  34.04,2.41 0 top
S2  11.18,2.41 0 top
S3  40.26,4.06 90 top
S4  53.72,4.06 90 top
S5  52.32,27.56 0 top
TP1  5.08,26.42 90 top
TP2  5.08,23.88 90 top
TP3  5.08,21.34 90 top
TP4  5.08,18.8 90 top
TP5  5.08,16.26 90 top
TP6  5.08,13.72 90 top
TP7  5.08,11.18 90 top
TP8  5.08,8.64 90 top
TP9  5.08,6.1 90 top
TP10  5.08,3.56 90 top
TP11  45.72,26.42 90 top
TP12  45.72,23.88 90 top
TP13  45.72,21.34 90 top
TP14  45.72,18.8 90 top
TP15  45.72,16.26 90 top
TP16  45.72,13.72 90 top
TP17  45.72,11.18 90 top
TP18  45.72,8.64 90 top
TP19  45.72,6.1 90 top
TP20  45.72,3.56 90 top
TP21  51.05,19.81 0 bottom
TP22  51.05,18.67 0 bottom
TP23  51.05,17.53 0 bottom
TP24  51.05,16.38 0 bottom
TP25  51.05,13.59 0 top
TP26  51.05,11.43 0 top
TP27  55.5,8.38 0 top
TP28  57.15,8.38 0 top
TP29  60.33,8.38 0 top
U1  14.1,17.78 270 top
U2  14.1,13.34 0 top
U3  14.1,7.62 90 top
U4  14.61,22.99 270 top
U5  25.4,14.99 270 top
U6  52.58,19.49 270 top
U$1  1.27,1.27 0 top
U$2  3.84,26.42 0 top
U$3  3.84,23.88 0 top
U$4  3.84,21.34 0 top
U$5  3.84,18.8 0 top
U$6  3.84,16.26 0 top
U$7  3.84,13.72 0 top
U$8  3.84,11.18 0 top
U$9  3.84,8.64 0 top
U$10  3.84,6.1 0 top
U$11  3.84,3.56 0 top
U$12  [ANAREN_LOGO_SCALE_0.2]  33.66,27.3 0 top
U$13  45.72,28.57 0 top
U$14  46.96,26.42 0 top
U$15  46.96,23.88 0 top
U$16  46.96,21.34 0 top
U$17  46.96,18.8 0 top
U$18  46.96,16.26 0 top
U$19  46.96,13.72 0 top
U$20  46.96,11.18 0 top
U$21  46.96,8.64 0 top
U$22  46.96,6.1 0 top
U$23  46.96,3.56 0 top
U$24  [LAUNCHPAD_HALF_ROCKET_SCALE_0.5]  66.04,0.76 0 top
U$25  [AIR_LOGO_SCALE_0.1]  69.72,25.4 270 top
U$100  [ANAREN_LOGO_SCALE_0.3]  69.6,1.02 90 bottom
U$101  [AIR_LOGO_SCALE_0.15]  66.8,23.11 90 bottom
U$102  [ESD_LOGO_SCALE_0.2]  64.01,12.19 90 bottom
U$103  [PB-FREE_LOGO_SCALE_1.0]  34.29,4.83 0 bottom
Y1  60.2,22.1 0 top

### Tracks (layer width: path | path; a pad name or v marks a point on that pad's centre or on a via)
CFG0  (via drill 0.25)
  Top 0.203: U6.20_GIO2 53.8,12.49 v53.85,12.45
  Bottom 0.203: v53.85,12.45 55.63,12.45 56.39,13.21 JP100.C
CFG1  (via drill 0.25)
  Top 0.203: v57.15,18.8 57.15,20.07 U6.9_GIO13
  Bottom 0.203: JP101.C 56.39,18.03 v57.15,18.8
CURRENT
  Top 0.203: U4.B2 15.93,22.79 JP2.1
D1,2_!EN
  Top 0.203: 21.34,2.16 24.77,2.16 27.18,4.57 30.73,4.57 32.77,6.6 38.23,6.6 38.23,6.24 S3.8 | 21.34,2.16 14.99,2.16 14.73,1.91 14.73,1.42 D1.2 | D2.2 21.32,2.14 21.34,2.16
D3,4_EN
  Top 0.203: D4.1(+) 13.67,19.98 13.97,19.68 17.53,19.68 19.18,18.03 19.18,10.92 20.45,9.65 22.73,9.65 24.77,7.62 30.61,7.62 31.11,8.13 41.15,8.13 42.16,7.11 S3.5 42.16,4.83 41.4,4.06 38.23,4.06 37.34,3.17 37.34,2.03 36.45,1.14 31.5,1.14 31.24,1.4 R14.1
GND  (via drill 0.25)
  Top 0.203: 52.7,10.49 U6.22_GND 51.64,10.49 51.44,10.29 v51.44,9.6 | 14.1,7.49 U3.B1 14.1,6.99 | 51.18,18.54 TP22.P$1 51.23,18.49 U6.14_USBP | C7.P$1 C8.P$1 60.71,23.51 v60.71,24.51 | C2.P$1 16.46,14.29 U2.6 15.1,15.22 v15.11,15.24 | S2.2 11.68,2.41 v11.18,1.91 | S1.2 34.67,2.41 v34.04,3.05 | S3.1 v38.35,3.17 | C9.P$2 62.68,7.81 62.99,7.49 v63.49,7.49 | v65.15,11.18 65.17,11.16 U6.34_GND 65.22,9.85 C10.P$2 | v65.15,18.8 65.15,20.07 | 65.15,20.07 U6.1_GND | 65.15,20.07 v65.15,21.4 65.19,21.45 D9.2 D8.2 | U6.3_GND 63.17,18.82 v63.15,18.8 | 16.63,18.03 U1.7 14.35,18.03 U1.9 13.85,18.03 U1.2 11.94,18.03 | 16.63,18.03 C3.P$2 | 16.63,18.03 17.14,18.03 v17.53,18.41 | U6.12_GND 54.17,18.86 v54.23,18.8 | J101.1 13.34,23.62 14.17,22.79 U4.B1 14.4,22.53 | U1.1 11.94,18.53 11.94,18.54 | U1.4 11.94,17.03 11.94,17.02 | U1.3 11.81,17.53
  Top 0.254: U3.A2 v12.7,7.62 | v9.65,7.62 C1.P$1
  Top 0.508: U$14.P2 J2.10
  Bottom 0.203: JP100.1 54.86,14.05 v54.86,14.99 54.86,15.93 JP101.2
  Bottom 0.254: v12.7,7.62 v9.65,7.62
  other vias: 1.4,25.15 1.4,28.57 46.99,1.32 63.12,21.34 58.67,11.18 11.94,13.97 56.64,24.89 25.4,23.88 25.4,26.42 24.77,5.46 24.77,3.56 43.18,26.42 43.18,23.88 43.18,21.34 43.18,18.8 43.18,16.26 43.18,13.72 43.18,11.18 43.18,8.64 43.18,1.4 33.02,23.24 33.02,20.7 33.15,18.16 33.02,15.62 33.02,13.21 25.4,21.97 25.4,14.99 7.49,19.05 7.49,15.75 7.49,11.43 7.49,22.86 19.43,1.4 19.68,20.7 57.15,1.47 18.67,7.37 51.69,4.19 20.32,27.81 52.32,27.56 33.02,10.54 58.55,22.23 35.56,5.59 50.04,4.19 12.06,16.51 63.37,1.47
  pour L2_GND: 10.16,1.12 1.5,1.12 arc-90 1.12,1.5 1.12,28.47 arc-90 1.5,28.85 64.97,28.85 arc-90 65.35,28.47 65.35,1.5 arc-90 64.97,1.12 10.19,1.12 10.19,3.68 18.03,3.68 18.03,11.56 10.16,11.56
  pour Top: 11.94,9.65 16.26,9.65 16.26,5.33 11.94,5.33
  pour Bottom: 11.94,9.65 16.26,9.65 16.26,5.33 11.94,5.33
  pour Top (rank 2): 10.16,1.12 1.5,1.12 arc-90 1.12,1.5 1.12,28.47 arc-90 1.5,28.85 64.97,28.85 arc-90 65.35,28.47 65.35,1.5 arc-90 64.97,1.12 10.19,1.12 10.19,3.68 18.03,3.68 18.03,11.56 10.16,11.56
  pour Bottom (rank 2): 10.16,1.12 1.5,1.12 arc-90 1.12,1.5 1.12,28.47 arc-90 1.5,28.85 64.97,28.85 arc-90 65.35,28.47 65.35,1.5 arc-90 64.97,1.12 10.19,1.12 10.19,3.68 18.03,3.68 18.03,11.56 10.16,11.56
GPIO0
  Top 0.203: U6.31_HGM 62.17,9.46 61.98,9.27 61.98,7.87 63.12,6.73 63.12,4.45 J5.4 61.21,2.54 61.21,2.03 60.45,1.27 58.42,1.27 55.75,3.94 53.21,3.94 51.82,5.33 S4.8
GPIO1
  Top 0.203: S4.7 53.09,5.21 53.85,4.45 55.88,4.45 58.55,1.78 60.2,1.78 60.58,2.16 60.58,4.06 61.21,4.7 61.21,5.08 J5.3 61.85,6.99 61.17,7.67 U6.30_GND
GPIO2
  Top 0.203: U6.25_BCLK 56.17,9.36 56.26,9.27 56.26,8 56.77,7.49 60.07,7.49 60.58,6.99 60.58,4.83 60.2,4.45 59.31,4.45 | S4.6 54.36,5.33 54.74,4.95 57.78,4.95 58.29,4.45 59.31,4.45 | J5.6 59.31,4.45
GPIO3
  Top 0.203: U6.23_RSTN 54.17,8.44 55.63,6.99 S4.5 55.63,5.97 55.88,5.71 J5.5
LED1
  Top 0.203: R9.1 D1.1
LED2
  Top 0.203: D2.1 R11.1
LED3
  Top 0.203: R14.2 D3.1
LED4
  Top 0.203: D4.2(-R) 10.85,21.38 R5.1
LED5
  Top 0.203: R8.1 14.61,20.45 D4.4(-G)
LED6
  Top 0.203: R7.1 14.61,21.46 D4.3(-B)
LGT_EN
  Top 0.203: S3.6 40.89,7.11 40.39,7.62 31.5,7.62 30.99,7.11 24.26,7.11 23.75,7.62 20.45,7.62 18.67,9.4 18.67,11.68 18.03,12.32 17.14,12.32 16.51,12.95 C2.P$2 16.4,13.34 U2.5
LP_VCC
  Top 0.203: U4.A1 14.4,24.13 R6.2
  Top 0.508: J1.1 U$2.P1
  Top 0.762: R6.2 14.12,26.32 14.22,26.42
  Top 1.016: D5.P$2 14.22,26.42 JP1.1
  pour L3_PWR: 1.12,25.78 1.12,28.47 arc-90 1.5,28.85 15.24,28.85 15.24,25.78
MODULE_DC
  Top 0.203: U6.7_SDA 59.17,20.71 57.78,22.1 57.78,28.19 58.29,28.7 61.72,28.7 J4.3
MODULE_DD  (via drill 0.25 pad 0.25)
  Top 0.203: U6.8_GIO12 58.04,20.22 58.04,20.95 v57.66,21.34 | v59.94,24.51 59.94,24.64 60.58,25.27 61.59,25.27 J4.4
  Bottom 0.203: v59.94,24.51 57.66,22.23 v57.66,21.34
MRDY  (via drill 0.25)
  Top 0.203: U6.28_AD1 59.17,8.88 v58.93,8.64
  Bottom 0.203: v58.93,8.64 58.93,8.89 58.55,9.27 55.24,9.27 50.8,4.83 50.8,3.81 49.4,2.41 43.81,2.41 42.29,3.94 33.02,3.94 31.11,2.03 26.8,2.03 25.4,3.43 25.4,9.91 25.15,10.16 JP108.C
MRST  (via drill 0.25)
  Top 0.203: U6.32_IOVDD 63.12,9.95 63.12,10.92 62.87,11.18 v62.36,11.18 | v54.1,22.61 54.1,23.4 R19.2 C6.P$1 55.37,23.51
  Bottom 0.203: J4.7 59.18,28.7 58.29,28.7 54.1,24.51 v54.1,22.61 54.1,21.37 JP102.2 56.05,21.34 62.36,15.02 v62.36,11.18 61.47,10.29 R100.1 54.09,11.06 52.83,12.32 50.55,12.32 49.4,11.18 49.4,10.54 48.77,9.91 39.37,9.91 J3.12
N$1  (via drill 0.25)
  Top 0.203: v55.63,3.17 S4.4 | v62.36,24.51 62.36,23.52 R20.2
  Bottom 0.203: v55.63,3.17 55.63,4.19 58.42,6.99 60.83,6.99 63.5,9.65 63.5,17.78 63.75,18.03 63.75,23.11 v62.36,24.51
N$2  (via drill 0.25)
  Top 0.203: v54.36,3.17 S4.3 | v62.36,21.34 62.36,22.45 R21.2
  Bottom 0.203: v54.36,3.17 54.36,3.56 58.29,7.49 60.71,7.49 62.99,9.78 62.99,17.78 62.36,18.41 v62.36,21.34
N$3
  Top 0.203: S4.2 53.09,2.79 52.7,3.17 50.8,3.17 49.91,2.29 45.59,2.29 45.24,1.93 R16.2
N$4
  Top 0.203: S4.1 51.82,1.78 51.56,1.52 48.94,1.52 R17.2
N$5
  Top 0.203: U6.6_SCL 60.17,21.11 59.59,21.69 59.59,21.97 Y1.1 59.46,22.45 59.04,22.87 C7.P$2
N$6
  Top 0.203: R12.2 24.92,20.04 D6.1
N$7
  Top 0.203: R13.2 24.92,9.94 D7.1
N$8
  Top 0.203: 14.35,23.62 14.1,23.88
N$9
  Top 0.203: 14.86,23.62 15.11,23.88
N$11
  Top 0.203: R3.2 R4.2 11.15,18.51 11.62,18.99 11.81,19.18 14.86,19.18 15.51,18.53 U1.8 15.86,18.53 16.13,18.8 16.62,18.8 C3.P$1
N$14
  Top 0.203: R21.1 D9.1
N$15
  Top 0.203: R20.1 D8.1
N$16
  Top 0.203: U6.13_USBM 52.51,19.56 51.31,19.56 TP21.P$1
  Bottom 0.508: JP104.P2 50.75,20.12 TP21.P$1
N$17
  Top 0.203: U6.15_CSN 52.55,17.53 TP23.P$1
  Bottom 0.508: JP103.P2 50.75,17.83 TP23.P$1
N$18
  Top 0.203: R19.1 R18.2 52.04,24.67 50.62,26.08 S5.1
N$19
  Top 0.203: U$2.P2 4.19,26.42
  Top 0.508: 4.19,26.42 TP1.1
N$24
  Top 0.508: U$6.P2 TP5.1
N$25
  Top 0.508: U$7.P2 TP6.1
N$26
  Top 0.508: U$8.P2 TP7.1
N$27
  Top 0.508: U$9.P2 TP8.1
N$28
  Top 0.508: U$10.P2 TP9.1
N$29
  Top 0.508: U$11.P2 TP10.1
N$30
  Top 0.508: U$14.P1 TP11.1
N$31
  Top 0.508: U$15.P1 TP12.1
N$32
  Top 0.508: U$16.P1 TP13.1
N$33
  Top 0.508: U$17.P1 TP14.1
N$34
  Top 0.508: U$18.P1 TP15.1
N$35
  Top 0.508: U$19.P1 TP16.1
N$36
  Top 0.508: U$20.P1 TP17.1
N$37
  Top 0.508: U$21.P1 TP18.1
N$38
  Top 0.508: U$22.P1 TP19.1
N$39
  Top 0.508: U$23.P1 TP20.1
N$40
  Top 0.203: U6.16_SCLK 51.17,16.49 TP24.P$1
N$42
  Top 1.016: J101.2 9.65,25.77 D5.P$1
P1.0/LED1  (via drill 0.25)
  Top 0.203: v18.41,1.4 R9.2
  Top 0.508: U$3.P1 J1.2
  Bottom 0.203: v18.41,1.4 18.16,1.14 2.79,1.14 1.14,2.79 1.14,22.48 J1.2 3.81,25.15 19.81,25.15 21.08,23.88 U5.2
P1.1/RXD
  Top 0.508: J1.3 U$4.P1
  Bottom 0.203: J1.3 3.43,22.23 3.81,22.61 6.86,22.61 8.13,21.34 U5.3
P1.2/TXD
  Top 0.508: J1.4 U$5.P1
  Bottom 0.203: J1.4 3.81,20.07 7.37,20.07 7.87,19.56 20.32,19.56 21.08,18.8 U5.4
P1.3/S2
  Top 0.203: J1.5 3.81,14.99 6.86,14.99 8.26,13.59 R1.1 9.48,2.9 S2.1
  Top 0.508: U$6.P1 J1.5
  Bottom 0.203: J1.5 3.81,17.53 6.86,17.53 8.51,15.88 20.45,15.88 20.83,16.26 U5.5
P1.4/CUR/MRDY/EXT_!CS  (via drill 0.25)
  Top 0.203: v23.88,21.34 23.88,15.49 22.1,13.72 U5.6
  Top 0.508: J1.6 U$7.P1
  Bottom 0.203: J3.2 36.83,25.15 33.53,25.15 30.99,22.61 23.88,22.61 | 23.88,22.61 19.78,22.61 JP2.2 | J1.6 3.81,14.99 6.86,14.99 7.24,14.61 20.19,14.61 21.08,13.72 U5.6 23.37,13.72 24.38,12.7 JP108.2 | v23.88,21.34 23.88,22.61
P1.5/SCLK
  Top 0.203: U6.17_MOSI 49.4,15.49 48.9,14.99 39.37,14.99 J3.8 36.83,14.99 33.02,14.99 30.73,12.7 23.62,12.7 22.1,11.18 U5.7
  Top 0.508: U$8.P1 J1.7
  Bottom 0.203: J1.7 3.81,12.45 6.86,12.45 7.75,13.34 17.02,13.34 19.18,11.18 U5.7
P1.6/MISO/LED2  (via drill 0.25)
  Top 0.203: J2.4 46.99,9.91 30.99,9.91 29.72,11.18 U5.14 | U6.10_PA 56.17,18.83 v56.13,18.8 | R11.2 25.02,1.4 v27.56,3.94
  Top 0.508: J2.4 U$20.P2
  Bottom 0.203: v27.56,3.94 27.56,10.03 28.7,11.18 | 28.7,11.18 U5.14 | 28.7,11.18 27.56,12.32 27.56,14.22 28.07,14.73 30.86,14.73 31.11,14.99 39.12,14.99 39.37,15.24 39.37,17.53 J3.6 | 56.01,18.8 v56.13,18.8 51.82,14.48 50.8,14.48 49.4,13.08 49.4,12.32 J2.4
P1.6/MISO/SCL/LED1
  Top 0.203: U6.5_VBAT 61.06,20.2 61.06,21.97 Y1.2 60.94,22.45 61.48,23 C8.P$2
P1.7/MOSI  (via drill 0.25)
  Top 0.203: J3.4 36.83,20.07 32.89,20.07 30.35,17.53 28.07,17.53 27.18,16.64 27.18,15.24 28.7,13.72 U5.15 | U6.11_LNA 55.17,18.85 v55.12,18.8
  Top 0.508: U$19.P2 J2.5
  Bottom 0.203: v55.12,18.8 51.94,15.62 50.16,15.62 J2.5 46.99,12.45 30.99,12.45 29.72,13.72 U5.15
P2.0/MODULE_SS  (via drill 0.25)
  Top 0.203: v23.37,10.92 24.64,12.19 33.53,12.19 33.78,12.45 36.83,12.45 J3.10 39.37,12.45 48.77,12.45 50.82,14.49 U6.18_MISO
  Top 0.508: U$9.P1 J1.8
  Bottom 0.203: J1.8 3.81,7.37 6.1,7.37 9.78,3.68 17.91,3.68 19.94,5.71 19.94,7.49 21.08,8.64 U5.8 23.37,8.64 | 23.37,8.64 24.31,8.64 JP108.1 | v23.37,10.92 23.37,8.64
P2.1/LED4
  Top 0.203: J1.9 1.14,7.49 1.14,21.84 1.91,22.61 6.86,22.61 8.99,20.48 R5.2
  Top 0.508: U$10.P1 J1.9
  Bottom 0.203: J1.9 3.81,4.83 6.86,4.83 8.51,3.17 18.16,3.17 21.08,6.1 U5.9
P2.2/SRDY
  Top 0.508: U$11.P1 J1.10
  Bottom 0.203: J1.10 3.81,2.29 6.86,2.29 7.24,2.67 20.19,2.67 21.08,3.56 U5.10 22.1,3.56 24.13,1.52 31.62,1.52 32.38,2.29 JP105.2
P2.3/SDA  (via drill 0.25)
  Top 0.203: v42.8,4.83 46.99,4.83 J2.1
  Top 0.508: U$23.P2 J2.1
  Bottom 0.203: JP106.1 v42.8,4.83
P2.4/SCL/LED3
  Top 0.508: U$22.P2 J2.2
  Bottom 0.203: J2.2 46.99,4.83 43.73,4.83 JP107.1
P2.5/LED5
  Top 0.203: J2.3 46.99,7.37 43.18,7.37 41.91,8.64 U5.13 24.77,8.64 23.24,10.16 20.57,10.16 19.68,11.05 19.68,18.29 17.53,20.45 R8.2
  Top 0.508: U$21.P2 J2.3
  Bottom 0.203: R100.2 49.91,10.29 J2.3
P2.6/LED6
  Top 0.203: J2.9 46.99,25.15 43.18,25.15 41.91,26.42 32.26,26.42 29.72,23.88 U5.19 28.7,23.88 27.43,22.61 19.81,22.61 18.67,21.46 R7.2
  Top 0.508: U$15.P2 J2.9
P2.7/MRST
  Top 0.203: J2.8 46.99,22.61 43.18,22.61 40.64,25.15 33.53,25.15 29.72,21.34 U5.18
  Top 0.508: U$16.P2 J2.8
  Bottom 0.203: JP102.1 J2.8
RST/S1  (via drill 0.25)
  Top 0.203: J2.6 48.26,16.38 47.12,17.53 33.78,17.53 32.51,16.26 31.62,16.26 | v32.13,4.19 32.13,2.62 S1.1 | U5.16 31.62,16.26 | R15.1 31.62,16.26 | 31.62,16.26 C5.P$1
  Top 0.508: U$18.P2 J2.6
  Bottom 0.203: v32.13,4.19 30.48,2.54 27.18,2.54 26.16,3.56 26.16,14.61 27.81,16.26 U5.16
SCL  (via drill 0.25)
  Top 0.203: U5.12 24.26,6.1 23.24,7.11 20.32,7.11 18.16,9.27 18.16,11.43 17.91,11.68 v14.1,11.68 14.1,14.35 | U3.B3 v14.1,9.02 | D3.2 27.87,1.84 28.57,2.54 30.48,2.54 31.24,3.3 31.24,4.32 32.89,5.97 v33.15,5.97 | 14.1,14.35 14.1,15.49 14.48,15.88 17.78,15.88 | U1.6 16.12,17.53 16.38,17.27 v16.64,17.27 17.14,17.27 17.78,16.64 17.78,15.88 | U2.1 14.03,14.29 14.1,14.35 | R10.2 17.78,15.88
  Top 0.508: U$4.P2 TP3.1
  Bottom 0.203: JP104.P1 49.71,19.51 49.15,20.07 43.18,20.07 40.64,22.61 34.54,22.61 34.04,22.1 34.04,18.8 | v14.1,9.02 v14.1,11.68 | 34.04,18.8 31.62,18.8 30.61,17.78 23.88,17.78 | 34.04,18.8 J3.5 | 23.88,17.78 17.14,17.78 v16.64,17.27 | TP3.1 6.86,21.34 8.13,20.07 22.86,20.07 23.88,19.05 23.88,17.78 | JP107.2 34.54,7.37 v33.15,5.97 29.34,5.97 U5.12
SDA  (via drill 0.25)
  Top 0.203: U3.C3 v15.49,9.02 | 16.38,16.51 v16.64,16.51 15.62,16.51 15.6,16.53 | U2.3 12,12.38 v11.94,12.32 11.3,12.95 11.3,14.29 11.28,14.32 | U1.5 15.6,16.53 | R2.2 11.28,14.32 | 11.28,14.32 13.46,16.51 15.57,16.51 15.6,16.53
  Top 0.508: U$5.P2 TP4.1
  Bottom 0.203: 4.45,18.8 TP4.1 6.86,18.8 8.51,17.14 15.24,17.14 15.88,16.51 v16.64,16.51 17.27,16.51 18.03,17.27 30.35,17.27 30.99,16.64 30.99,16.26 | v15.49,9.02 15.49,11.68 14.86,12.32 v11.94,12.32 | JP103.P1 49.71,17.22 49.4,17.53 43.18,17.53 40.64,20.07 37.08,20.07 36.83,19.81 36.83,17.53 J3.7 30.99,16.26 | 30.99,16.26 30.99,15.62 30.61,15.24 27.69,15.24 26.92,14.48 26.92,3.68 27.3,3.3 28.96,3.3 U5.11 29.72,3.56 30.99,4.83 JP106.2
SRDY  (via drill 0.25)
  Top 0.203: U6.27_AD0 v58.17,8.64
  Bottom 0.203: 58.17,8 52.07,1.91 43.69,1.91 43.31,2.29 JP105.1 | J3.11 38.1,8.64 41.91,8.64 43.18,7.37 52.7,7.37 55.12,9.78 58.93,9.78 59.56,9.14 59.56,8.38 59.18,8 58.17,8 | 58.17,8 v58.17,8.64
STLRS_GND
  Top 0.508: U$3.P2 TP2.1
TEMP/ROM_EN  (via drill 0.25)
  Top 0.203: S3.7 39.62,6.86 39.37,7.11 32.51,7.11 30.48,5.08 26.92,5.08 26.67,4.83 19.18,4.83 18.03,3.68 10.16,3.68 8.76,5.08 8.76,9.27 | C1.P$2 9.64,9.27 8.76,9.27 | 8.76,9.27 8.76,16 9.4,16.64 R3.1
  Top 0.254: U3.A3 v12.7,9.02 | v9.65,10.16 C1.P$2
  Bottom 0.254: v12.7,9.02 10.16,9.02 9.65,9.53 v9.65,10.16
TEST
  Top 0.203: J2.7 46.99,20.07 43.18,20.07 40.64,22.61 33.53,22.61 29.72,18.8 U5.17
  Top 0.508: U$17.P2 J2.7
TP_EN
  Top 0.203: U6.19_GIO1 51.15,13.49 TP25.P$1
TP_HGM
  Top 0.203: U6.24_MCLK 55.17,8.71 TP27.P$1
TP_P02
  Top 0.203: U6.29_GIO9/AD2 60.17,8.54 TP29.P$1
TP_P05
  Top 0.203: U6.26_WCLK 57.17,8.4 TP28.P$1
TP_PAEN
  Top 0.203: U6.21_GIO3 51.12,11.49 TP26.P$1
VDD  (via drill 0.25, 0.25 pad 0.25)
  Top 0.203: v32.38,17.78 31.65,17.78 R15.2 | R1.2 7.4,1.94 v7.24,1.78 | R2.1 v10.41,12.32 | C4.P$1 21.98,26.81 U5.1 | R10.1 18.44,13.36 v18.54,13.46 | R12.1 v26.92,18.8 | R13.1 v27.56,11.18 | R18.1 v50.16,23.5 | R4.1 v9.27,17.91
  Top 0.254: S3.2 S3.3 S3.4 v42.16,3.17
  L3_PWR 0.635: U5.1 21.59,25.15
  Bottom 0.203: JP101.1 58.04,15.95 v58.04,14.99 58.04,14.02 JP100.2
  Bottom 0.254: J4.2 62.87,25.27 59.05,25.27 v56.26,22.48
  pour L3_PWR (rank 2): 10.16,1.12 1.5,1.12 arc-90 1.12,1.5 1.12,28.47 arc-90 1.5,28.85 64.97,28.85 arc-90 65.35,28.47 65.35,1.5 arc-90 64.97,1.12 10.19,1.12 10.19,3.68 18.03,3.68 18.03,11.56 10.16,11.56
VDD_RADIO  (via drill 0.25 pad 0.25)
  Top 0.203: C9.P$1 C10.P$1 64.43,9.11 64.17,9.36 U6.33_VDD | U4.A2 14.8,24.13 R6.1
  Top 0.559: v64.19,11.18 64.19,9.92 U6.33_VDD
  Top 0.762: R6.1 15.09,24.36 15.62,24.89 17.21,24.89 JP1.3
  pour L3_PWR: 18.21,28.85 64.97,28.85 arc-90 65.35,28.47 65.35,10.92 63.5,10.92 63.25,11.18 63.25,16.51 53.98,25.78 18.21,25.78

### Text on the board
tPlace: J1 | 1 | C | 2 | J2 | GND | VCC | GND | P2.6 | AIR MODULE | RESET | POWER | P1.0 | CSNX | VDD | P2.7 | P1.1 | RGB | LED | SCL | MOSI | TEST | P1.2 | MISO | SDA | RST | EEPROM | P1.3 | GND | SCLK | P1.7 | P1.4 | RGB | CSNR | SENSOR | SRDY | P1.6 | P1.5 | MRST | P2.5 | SENS | P2.0 | SENSOR | GPIO | D1/2 | TEMP | RGB | D3/4 | P2.4 | 0 | 1 | 2 | 3 | IO 3 | IO 1 | GND | TEMP | P2.1 | MCU | P2.3 | IR | RESET | P2.2 | IO 2 | IO 0 | VDD
bPlace: J1 | 66931-0003 | J2 | VCC | GND | P1.0 | CSNX | GND | P2.6 | P1.1 | MOSI | EXT PWR | VDD | P1.2 | (+) | (-) | MISO | P2.7 | SCL | TEST | P1.3 | SCLK | 2 | C | 1 | RST | P1.4 | SDA | CSNR | EN | DEVICE | GND | P1.7 | PAEN | ESD SENSITIVE | P1.5 | MRST | 1 | C | 2 | P2.0 | SRDY | P1.6 | P2.5 | P2.1 | IO 3 | IO 1 | GND | HGM | P2.2 | P2.4 | P2.3 | IO 2 | IO 0 | VDD
DrillLegend: LAYER-STACK
DrillLegend_01-02: 01-16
